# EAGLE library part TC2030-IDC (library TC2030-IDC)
CABLE ADAPTER 6 POS Source: Datasheet
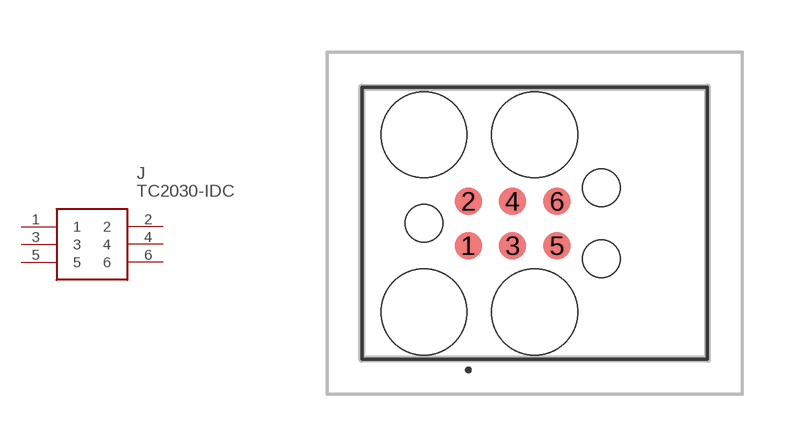
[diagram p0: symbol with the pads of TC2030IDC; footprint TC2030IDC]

Designator prefix J

## TC2030-IDC (Description: CABLE ADAPTER 6 POS; Height: 19mm; Manufacturer_Name: Tag Connect; Manufacturer_Part_Number: TC2030-IDC)  [TC2030IDC]
1  1
2  2
3  3
4  4
5  5
6  6

## Footprint TC2030IDC (pad centres in mm)
TC2030-IDC
smd 0.783 x 0.783: 1 -0.953,-0.635; 2 -0.953,0.635; 3 0.317,-0.635; 4 0.317,0.635; 5 1.588,-0.635; 6 1.588,0.635
hole 2.451 at -2.223,-2.54
hole 1.067 at -2.223,0
hole 2.451 at -2.223,2.54
hole 2.451 at 0.952,-2.54
hole 2.451 at 0.952,2.54
hole 1.067 at 2.857,-1.016
hole 1.067 at 2.857,1.016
